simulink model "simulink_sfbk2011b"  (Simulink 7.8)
settings: Solver=ode4  StartTime=0.0  StopTime=1  FixedStep=1e-2  RelTol=1e-3
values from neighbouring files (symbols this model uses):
  A = [-3 1; 2 -2]    [poleplace_acker.m]    (also in poleplace_ctrb.m)
  B = [2; 0]    [poleplace_acker.m]    (also in poleplace_ctrb.m)
  K1 = Kc1*Tc    [poleplace_ctrb.m]
  K2 = Kc2*Tc    [poleplace_ctrb.m]
  K3 = Kc3*Tc    [poleplace_ctrb.m]
  x0 = [0; 1]    [poleplace_ctrb.m]

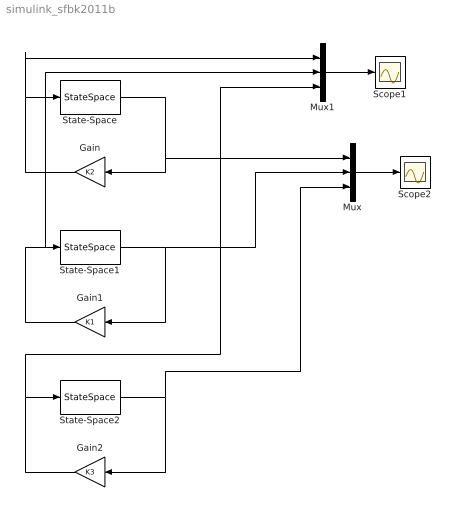
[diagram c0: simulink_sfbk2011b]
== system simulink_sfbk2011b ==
  Gain : Gain  Gain=K2  Multiplication=Matrix(K*u) (u vector)
  Gain1 : Gain  Gain=K1  Multiplication=Matrix(K*u) (u vector)
  Gain2 : Gain  Gain=K3  Multiplication=Matrix(K*u) (u vector)
  Mux : Mux  Inputs=3
  Mux1 : Mux  Inputs=3
  Scope1 : Scope
  Scope2 : Scope
  State-Space : StateSpace  A=A  B=B  C=eye(2)  D=zeros(2,1)  X0=x0
  State-Space1 : StateSpace  A=A  B=B  C=eye(2)  D=zeros(2,1)  X0=x0
  State-Space2 : StateSpace  A=A  B=B  C=eye(2)  D=zeros(2,1)  X0=x0
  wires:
  State-Space/1 -> Mux/1, Gain/1
  Gain/1 -> Mux1/1, State-Space/1
  Gain1/1 -> Mux1/2, State-Space1/1
  State-Space1/1 -> Mux/2, Gain1/1
  Gain2/1 -> Mux1/3, State-Space2/1
  State-Space2/1 -> Mux/3, Gain2/1
  Mux/1 -> Scope2/1
  Mux1/1 -> Scope1/1
